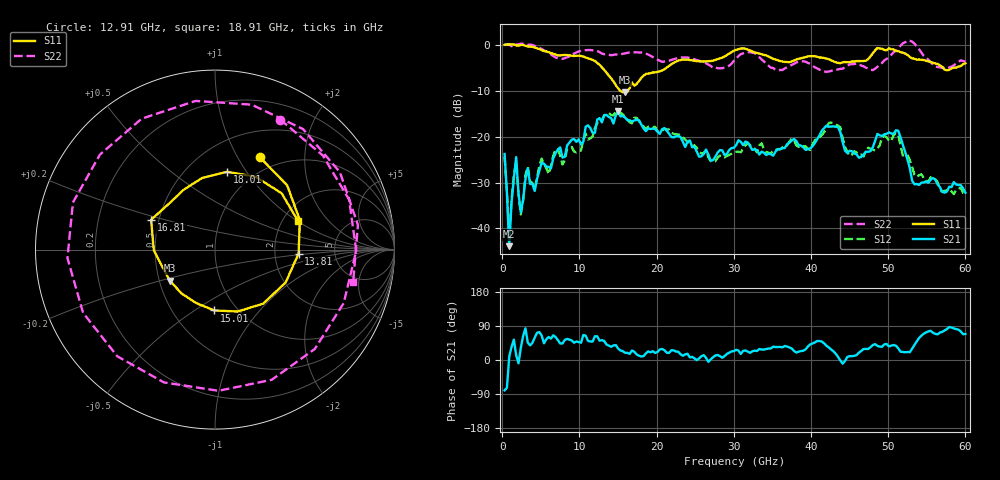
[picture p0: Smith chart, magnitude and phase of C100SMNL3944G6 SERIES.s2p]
! 12/11/2024 5:13:52 AM
! D:\C100SMNL3944G6 SERIES.S2P
! CHANNEL.1
! TR.MEASUREMENT
! CORRECTED.DATA
# GHZ S RI R 50.0
! FREQ.GHZ  S11RE  S11IM  S21RE  S21IM  S12RE  S12IM  S22RE  S22IM
!; PortSelection: Port_12
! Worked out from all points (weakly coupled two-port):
!   200 points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, 309.9 MHz to 60 GHz, reference 50 ohm
!   highest |S21| = -14.33 dB at 15.01 GHz (marker M1); lowest = -43.9 dB at 909.9 MHz (marker M2)
!   lowest |S11| = -10.3 dB at 15.91 GHz (marker M3), VSWR 1.88, Z = 28.4 - j10.8 ohm
!   |S11| at or under -10 dB: 15.3 GHz to 16.27 GHz (972.4 MHz wide, 6.16 % of centre)
!   |S22| runs from -5.8 to 1.0 dB; largest |S21 - S12| = 0.051
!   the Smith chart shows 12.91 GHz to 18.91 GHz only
!   S11 on the Smith chart (normalised r, x): 12.91 GHz: 0.81, +1.24; 13.81 GHz: 2.74, -0.15; 15.01 GHz: 0.79, -0.60; 16.81 GHz: 0.45, +0.18; 18.01 GHz: 0.76, +0.82; 18.91 GHz: 2.43, +1.01
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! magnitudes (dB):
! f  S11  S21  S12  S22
! 309.9 MHz  0.1  -23.8  -24.4  0.1
! 909.9 MHz  0.1  -43.9  -42.4  0.2
! 1.81 GHz  0.0  -24.4  -25.5  0.1
! 2.41 GHz  0.1  -36.5  -36.9  0.4
! 3.309 GHz  -0.3  -26.9  -26.4  0.1
! 4.209 GHz  -0.5  -31.8  -31.4  -0.1
! 5.109 GHz  -1.1  -25.7  -24.7  -0.8
! 10.51 GHz  -2.5  -21.1  -20.6  -1.1
! 12.91 GHz  -4.8  -16.8  -16.4  -1.8
! 13.81 GHz  -6.6  -15.7  -14.8  -2.1
! 15.01 GHz  -9.4  -14.3  -15.0  -2.1
! 15.91 GHz  -10.3  -15.7  -15.7  -1.8
! 16.81 GHz  -8.1  -16.6  -17.1  -1.6
! 18.01 GHz  -7.2  -17.3  -17.2  -1.6
! 18.91 GHz  -6.2  -18.2  -17.8  -2.0
! 20.41 GHz  -5.7  -19.4  -18.9  -3.4
! 30.3 GHz  -1.0  -21.8  -23.3  -2.9
! 40.2 GHz  -2.4  -22.1  -21.6  -4.5
! 42.6 GHz  -3.3  -17.8  -16.9  -5.6
! 50.1 GHz  -0.7  -19.0  -20.9  -2.5
! 53.4 GHz  -2.9  -30.4  -28.3  0.3
! 60 GHz  -4.0  -32.2  -32.4  -3.6
